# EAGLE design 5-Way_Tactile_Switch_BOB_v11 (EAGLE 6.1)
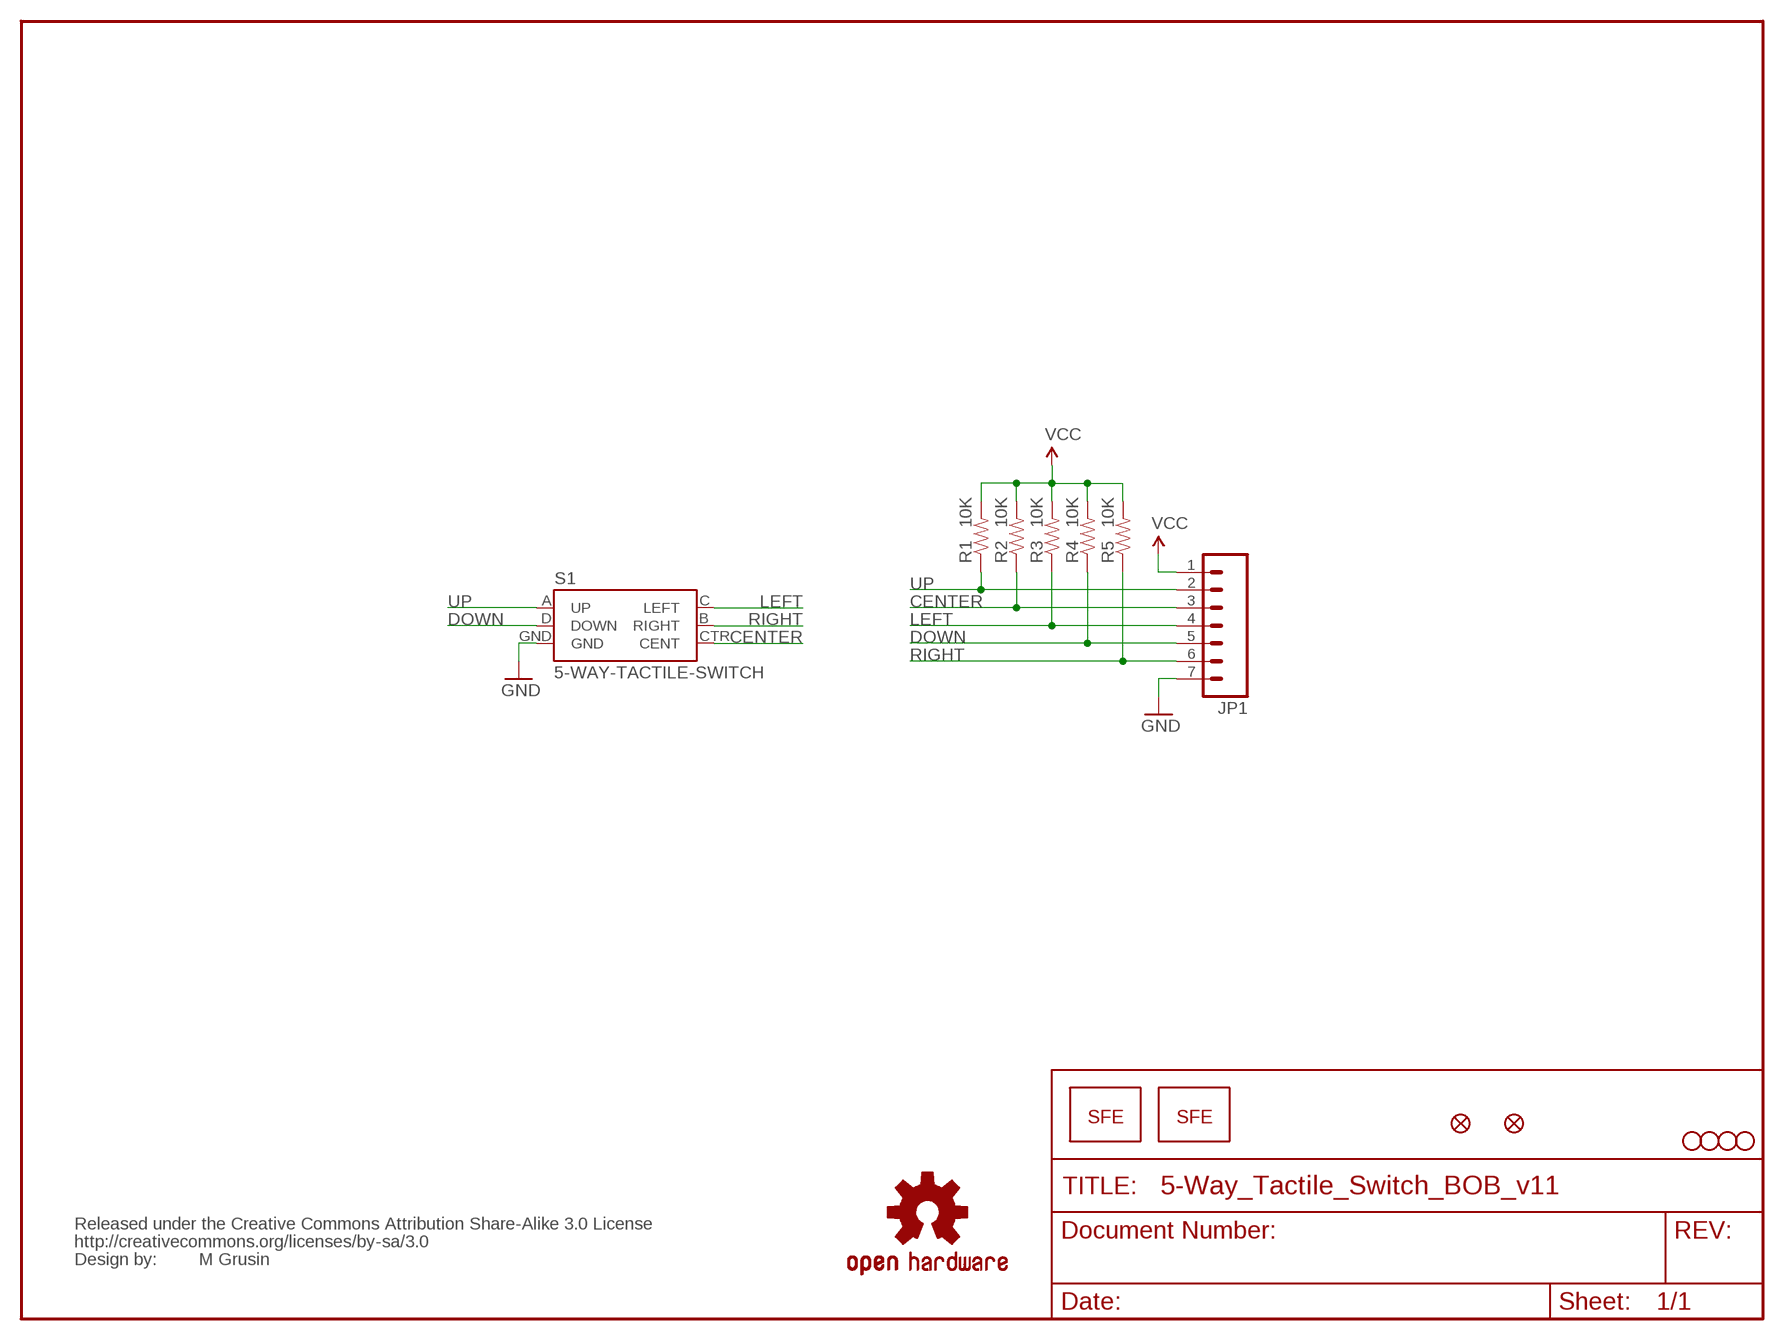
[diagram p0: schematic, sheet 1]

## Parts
JP1  M07  [1X07]
JP2  FIDUCIALUFIDUCIAL  [MICRO-FIDUCIAL]
JP3  STAND-OFF  [STAND-OFF]
JP4  STAND-OFF  [STAND-OFF]
JP5  STAND-OFF  [STAND-OFF]
JP6  STAND-OFF  [STAND-OFF]
JP7  FIDUCIALUFIDUCIAL  [MICRO-FIDUCIAL]
JP9  LOGO-SFESK  [SFE-LOGO-FLAME]
JP10  LOGO-SFENW2  [SFE-NEW-WEB]
R1  10K  RESISTOR0603-RES  [0603-RES]
R2  10K  RESISTOR0603-RES  [0603-RES]
R3  10K  RESISTOR0603-RES  [0603-RES]
R4  10K  RESISTOR0603-RES  [0603-RES]
R5  10K  RESISTOR0603-RES  [0603-RES]
S1  5-WAY-TACTILE-SWITCH  JOYSTICK_MINI  [JOYSTICK_MINI]
U$1  OSHW-LOGOS  [OSHW-LOGO-S]
U$2  CREATIVE_COMMONS  [CREATIVE_COMMONS]

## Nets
CENTER: JP1.3 R2.1 S1.CTR(CENT)
DOWN: JP1.5 R4.1 S1.D(DOWN)
GND: JP1.7 S1.GND
LEFT: JP1.4 R3.1 S1.C(LEFT)
RIGHT: JP1.6 R5.1 S1.B(RIGHT)
UP: JP1.2 R1.1 S1.A(UP)
VCC: JP1.1 R1.2 R2.2 R3.2 R4.2 R5.2

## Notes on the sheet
- M Grusin

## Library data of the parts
JP1 = SparkFun:M07: Header 7 Standard 7-pin 0.1" header. Use with straight break away headers (SKU : PRT-00116), right angle break away headers (PRT-00553), swiss pins (PRT-00743), machine pins (PRT-00117), and female headers (PRT-00115). NOTES ON THE VARIANTS LOCK and LOCK_LONGPADS... This footprint was designed to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
JP2 JP7 = SparkFun:FIDUCIAL: Fiducial Alignment Points
JP3-JP6 = SparkFun:STAND-OFF: Stand Off
JP9 JP10 = SparkFun:LOGO-SFE: Spark Fun Electronics PCB Logo
R1-R5 = SparkFun:RESISTOR: Resistor
S1 = SparkFun-Electromechanical:JOYSTICK_MINI: Small 5-way tactile joystick, COM-10063 4UCON SF303GJ26
U$1 = SparkFun:OSHW-LOGO: Open Source Hardware Logo This logo indicates the piece of hardware it is found on incorporates a OSHW license and/or adheres to the definition of open source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
U$2 = SparkFun:CREATIVE_COMMONS

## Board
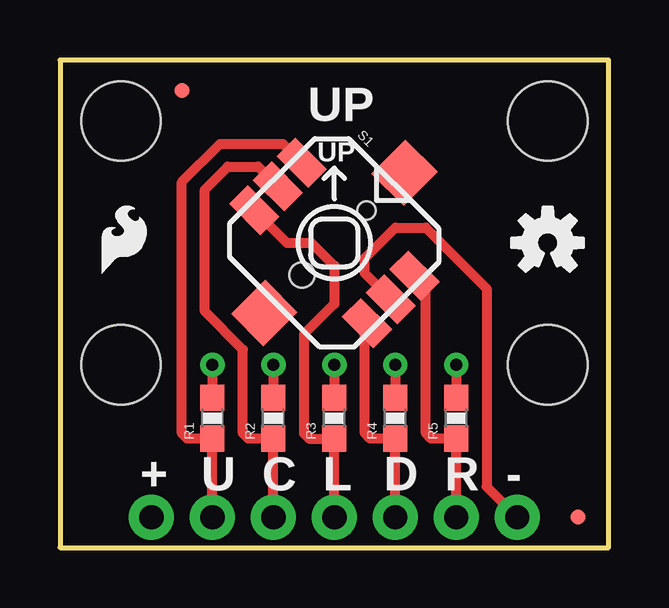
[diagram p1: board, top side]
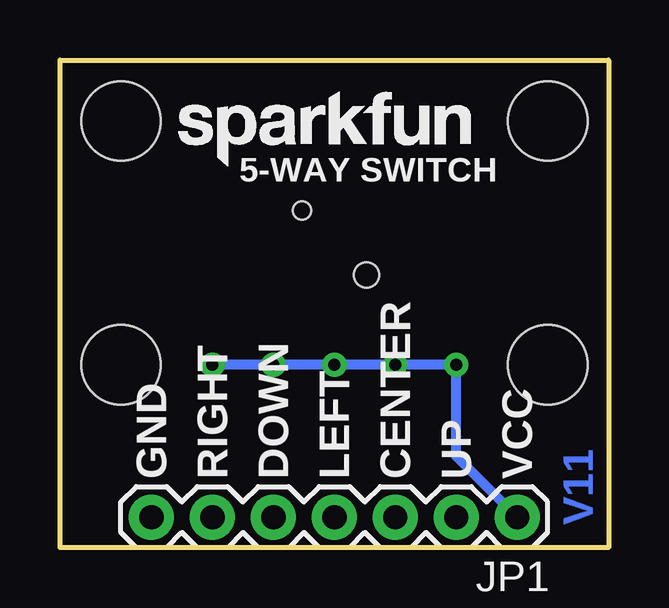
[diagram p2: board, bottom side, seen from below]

Size 22.86 x 20.32 mm. Coordinates in mm from the lower left corner, seen from the top.
Outline: 0,0 22.86,0 22.86,20.32 0,20.32 0,0
Copper layers (1*16): Top 0.035mm / dielectric 1.5mm / Bottom 0.035mm
Design rules: minimum track width 8mil, minimum drill 20mil, track to track 8mil, track to pad 8mil, pad to pad 8mil, via to via 8mil, smd to smd 8mil, copper to edge 8mil, drill to drill 8mil, minimum pad ring 12mil, minimum via ring 10mil, stop-mask expansion 4mil, vias tented up to drill 20mil, thermal gap 10mil

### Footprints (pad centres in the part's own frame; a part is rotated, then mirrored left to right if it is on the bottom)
1X07 = drill 1.016 pad 1.88: 1 0,0; 2 2.54,0; 3 5.08,0; 4 7.62,0; 5 10.16,0; 6 12.7,0; 7 15.24,0
MICRO-FIDUCIAL = smd 0.635 x 0.635: 1 0,0
STAND-OFF = hole 3.302: 0,0
0603-RES = smd 1.1 x 1: 1 -0.85,0; 2 0.85,0
JOYSTICK_MINI = smd 1.85 x 1.1: A -3.325,1.4; B 3.325,1.4; C -3.325,-1.4; CTR -3.325,0; D 3.325,-1.4; GND 3.325,0 | smd 1.9 x 2: NC 0,4.13; NC@0 0,-4.13 | hole 0.75: 0,1.9 | hole 1.05: 0,-1.9

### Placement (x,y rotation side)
JP1  3.81,1.27 180 bottom
JP2  21.59,1.27 0 top
JP3  20.32,17.78 0 top
JP4  20.32,7.62 0 top
JP5  2.54,17.78 0 top
JP6  2.54,7.62 0 top
JP7  5.08,19.05 0 top
JP9  1.75,11.43 0 top
JP10  17.94,15.88 0 bottom
R1  6.35,5.4 90 top
R2  8.89,5.4 90 top
R3  11.43,5.4 90 top
R4  13.97,5.4 90 top
R5  16.51,5.4 90 top
S1  11.43,12.7 315 top
U$1  20.32,12.7 0 top
U$2  not placed on the board

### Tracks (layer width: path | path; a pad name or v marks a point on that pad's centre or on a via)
CENTER
  Top 0.406: S1.CTR 8.26,15.88 6.99,15.88 6.03,14.92 6.03,9.84 7.62,8.26 7.62,4.76 7.83,4.55 R2.1 JP1.3
DOWN
  Top 0.406: S1.D 12.7,9.27 12.7,4.76 12.91,4.55 R4.1 JP1.5
GND
  Top 0.406: S1.GND 12.7,11.43 12.7,12.06 13.97,13.34 15.24,13.34 17.78,10.79 17.78,2.54 JP1.7
LEFT
  Top 0.406: S1.C 9.45,12.7 10.48,12.7 11.43,11.75 11.43,10.16 10.16,8.89 10.16,4.76 10.38,4.55 R3.1 JP1.4
RIGHT
  Top 0.406: JP1.6 R5.1 15.46,4.55 15.24,4.76 15.24,10.87 S1.B
UP
  Top 0.406: S1.A 9.28,16.83 6.67,16.83 5.08,15.24 5.08,4.76 5.29,4.55 R1.1 JP1.2
VCC  (via drill 0.51)
  Top 0.406: v6.35,7.62 R1.2 | v8.89,7.62 R2.2 | v11.43,7.62 R3.2 | v13.97,7.62 R4.2 | v16.51,7.62 R5.2
  Bottom 0.406: JP1.1 6.35,3.81 v6.35,7.62 v8.89,7.62 v11.43,7.62 v13.97,7.62 v16.51,7.62

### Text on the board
Bottom: V11
tPlace: UP | + | U | C | L | D | R | -
bPlace: 5-WAY SWITCH | VCC | UP | CENTER | LEFT | DOWN | RIGHT | GND
tValues: M Grusin
Document: 0.00" | 0.10" | 0.15" | 0.45" | 0.80" | 0.90" | 0.80" | 0.70" | 0.50" | 0.30" | 0.05" | 0.00"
